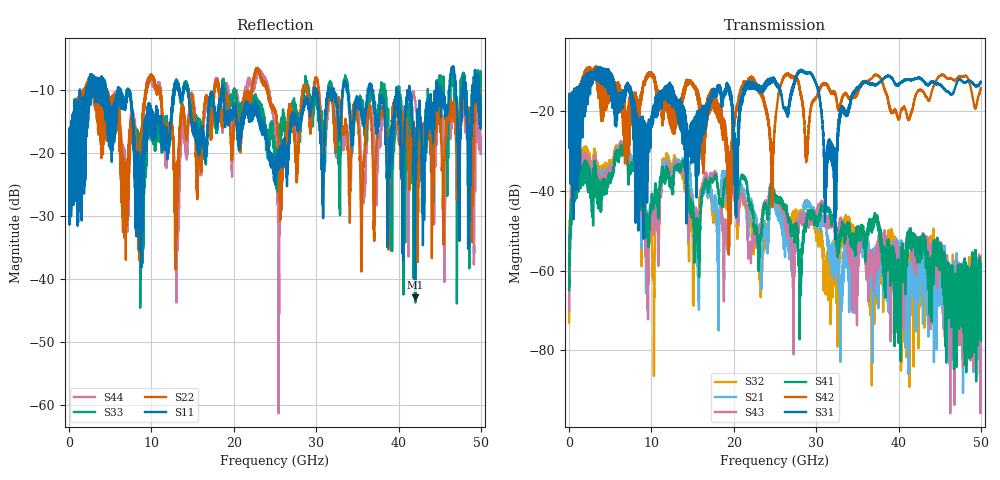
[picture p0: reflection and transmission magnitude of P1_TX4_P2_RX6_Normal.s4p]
!Keysight Technologies,N5225B,MY57041031,A.13.20.10
!Date: Friday, May 31, 2019 11:37:01
!Correction: S11(Full 4 Port(1,2,3,4))
!S12(Full 4 Port(1,2,3,4))
!S13(Full 4 Port(1,2,3,4))
!S14(Full 4 Port(1,2,3,4))
!S21(Full 4 Port(1,2,3,4))
!S22(Full 4 Port(1,2,3,4))
!S23(Full 4 Port(1,2,3,4))
!S24(Full 4 Port(1,2,3,4))
!S31(Full 4 Port(1,2,3,4))
!S32(Full 4 Port(1,2,3,4))
!S33(Full 4 Port(1,2,3,4))
!S34(Full 4 Port(1,2,3,4))
!S41(Full 4 Port(1,2,3,4))
!S42(Full 4 Port(1,2,3,4))
!S43(Full 4 Port(1,2,3,4))
!S44(Full 4 Port(1,2,3,4))
!S4P File: Measurements: <S11,S12,S13,S14>,
!<S21,S22,S23,S24>,
!<S31,S32,S33,S34>,
!<S41,S42,S43,S44>:
# Hz S  dB  R 50.0
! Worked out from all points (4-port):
!   5000 points, 10 MHz to 50 GHz, reference 50 ohm
!   strongest paths, dB at 10 MHz, 12.51 GHz, 25.01 GHz, 37.51 GHz, 50 GHz:
!     S31: -19.5, -17.6, -13.0, -13.1, -12.8
!     S42: -19.4, -16.8, -23.7, -11.2, -14.3
!     S41: -64.9, -38.6, -41.9, -47.9, -77.6
!     S43: -69.9, -36.4, -42.2, -57.5, -67.7
!     S21: -64.4, -37.0, -44.3, -61.8, -71.9
!     S32: -73.0, -34.8, -41.3, -56.8, -62.4
!   lowest |S11| = -42.9 dB at 42 GHz (marker M1), VSWR 1.01, Z = 49.3 + j0.123 ohm
!   |S11| at or under -10 dB: 7.331 GHz to 12.7 GHz (5.369 GHz wide, 53.6 % of centre); 14.37 GHz to 18.57 GHz (4.2 GHz wide, 25.5 % of centre); 18.74 GHz to 29.77 GHz (11.03 GHz wide, 45.5 % of centre)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
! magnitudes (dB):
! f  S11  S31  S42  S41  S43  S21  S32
! 10 MHz  -19.0  -19.5  -19.4  -64.9  -69.9  -64.4  -73.0
! 820 MHz  -17.7  -18.7  -17.3  -36.5  -34.3  -34.1  -32.0
! 6.74 GHz  -12.9  -15.5  -29.8  -27.6  -27.2  -26.9  -27.2
! 10.17 GHz  -17.1  -20.7  -11.4  -43.9  -51.2  -45.5  -60.0
! 11.92 GHz  -19.4  -17.6  -16.4  -34.5  -33.4  -32.5  -31.0
! 42 GHz  -42.9  -12.0  -16.7  -50.9  -55.4  -60.6  -60.6
! 50 GHz  -12.1  -12.8  -14.3  -77.6  -67.7  -71.9  -62.4
